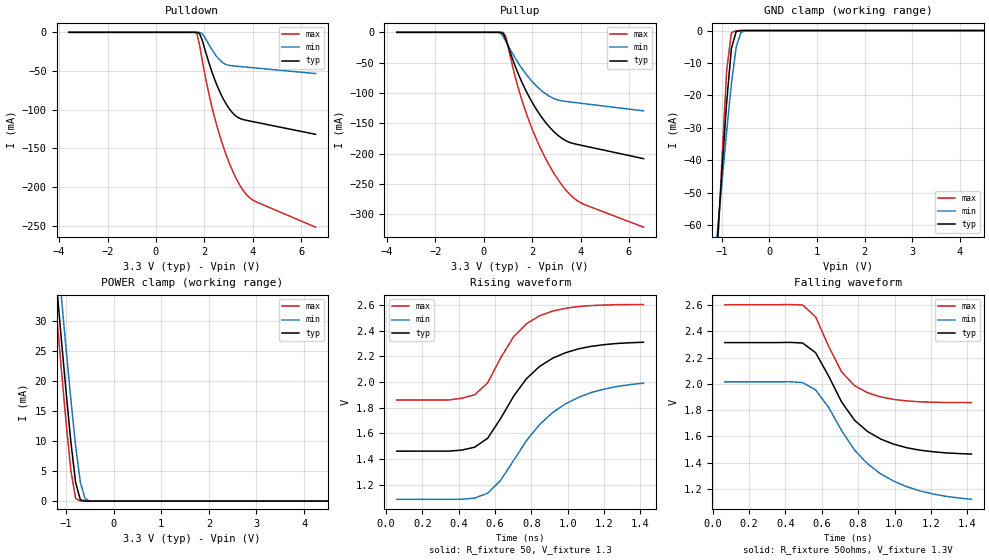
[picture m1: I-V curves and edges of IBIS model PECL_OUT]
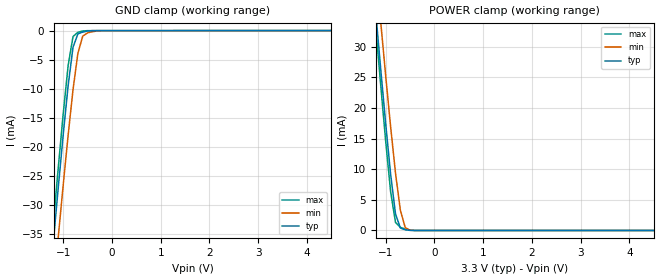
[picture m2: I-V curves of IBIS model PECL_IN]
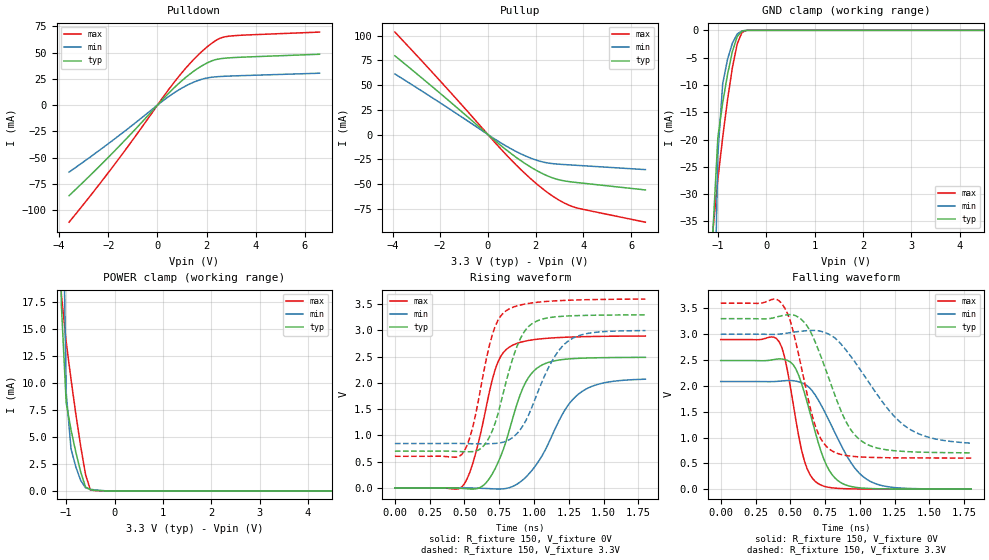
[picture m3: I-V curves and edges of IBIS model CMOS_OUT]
|   This file is an IBIS representation of the   |
|   Texas Instruments   |
|   CDCM1804   |
|   24-pin MLF Package   |
[IBIS Ver]   3.2
[File name]   cdcm1804.ibs
[File Rev]   0.4
[Date]   18th of Feb 2004
[Source]   file originated at Texas Instruments
[Notes]   The following information corresponds to the
|   CDCM1804 i/o buffers and input ESD structures.
|Revision log: 0.1, 06/03/2003 file released by TEXAS INSTRUMENTS.
|   1- initial version
|   0.2, 02/06/2004 file revised for CDCM1804
|   0.3, 02/17/2004 corrected Cin/Cout for PECL outputs,
|   corrected Vinl, Vinh for control input.
|   0.4, 02/18/2004 replaced GND clamp (referenced to VDD) by same
|   plot referenced to GND (0V).
|   Warnings for VT/IV voltage difference relate to truncated
|   VT plots to allow faster simulation frequency if
|   VT time delay is enabled, which is strongly recommended for
|   correct results of the differential PECL buffers. If this is not
|   required, some simulators require to completely disable use of
|   the VT table for better results. If you note problems with
|   differential cross point, it might point to this situation !
[Disclaimer]
(C) Copyright Texas Instruments Incorporated 2004
   All rights reserved
  Texas Instruments Incorporated hereby grants the user of this IBIS
model a non-exclusive, nontransferable license to use this IBIS model
under the following terms.  Before using this IBIS model, the user
should read this license.  If the user does not accept these terms,
the IBIS model should be returned to Texas Instruments within 30 days.
  The user is granted this license only to use the IBIS model and
is not granted rights to sell, load, rent, lease or license the IBIS
model in whole or in part, or in modified form to anyone other than
user.  User may modify the IBIS model to suit its specific applications
but rights to derivative works and such modifications shall belong to
Texas Instruments.
  This IBIS model is provided on an "AS IS" basis and Texas Instruments
makes absolutely no warranty with respect to the information contained
herein.  TEXAS INSTRUMENTS DISCLAIMS AND CUSTOMER WAIVES ALL WARRANTIES,
EXPRESS OR IMPLIED, INCLUDING WARRANTIES OF MERCHANTABILITY OR FITNESS
FOR A PARTICULAR PURPOSE. The entire risk as to quality and performance
is with the Customer. ACCORDINGLY, IN NO EVENT SHALL THE COMPANY BE LIABLE
FOR ANY DAMAGES, WHETHER IN CONTRACT OR TORT,INCLUDING ANY LOST PROFITS
OR OTHER INCIDENTAL, CONSEQUENTIAL, EXEMPLARY, OR PUNITIVE DAMAGES ARISING
OUT OF THE USE OR APPLICATION OF THE IBIS model provided in this package.
Further, Texas Instruments reserves the right to discontinue or make changes
without notice to any product herein to improve reliability, function, or
design. Texas Instruments does not convey any license under patent rights
or any other intellectual property rights, including those of third parties.
Contact Texas Instruments at ATTN: HPA Department,
12500 TI blvd, M/S 8730, Dallas, TX 75243
IBIS Open Forum disclaims all warranties. See DISCLAIM.TXT
in vhdl.org:/pub/IBIS/models for the full disclaimer.
[Copyright]   Copyright 2004, Texas Instruments, All Rights Reserved
[Component]   CDCM1804RTH
[Manufacturer]  Texas Instruments Incorporated
[Package]
|   TYP   MIN   MAX
R_pkg   0.260   0.150   0.310
L_pkg   1.150nH   0.220nH   1.370nH
C_pkg   0.041pF   0.027pF   0.047pF
[Pin]   signal_name   model_name   R_Pin   L_Pin   C_Pin
1   EN   CTRL_IN   0.167ohms   0.683nH   0.028pF
2   VDD   POWER   0.130ohms   0.600nH   0.080pF
3   IN   PECL_IN   0.285ohms   1.249nH   0.044pF
4   INB   PECL_IN   0.270ohms   1.176nH   0.041pF
5   VDD   POWER   0.130ohms   0.600nH   0.080pF
6   VBB   POWER   0.279ohms   1.221nH   0.044pF
7   VSS   GND   0.050ohms   0.220nH   0.240pF
8   VDD   POWER   0.130ohms   0.600nH   0.080pF
9   Y2   PECL_OUT   0.285ohms   1.250nH   0.044pF
10   Y2B   PECL_OUT   0.270ohms   1.177nH   0.041pF
11   VDD   POWER   0.130ohms   0.600nH   0.080pF
12   Y3   CMOS_OUT   0.302ohms   1.331nH   0.045pF
13   VDD   POWER   0.130ohms   0.600nH   0.080pF
14   VDD   POWER   0.130ohms   0.600nH   0.080pF
15   Y1   PECL_OUT   0.270ohms   1.176nH   0.041pF
16   Y1B   PECL_OUT   0.268ohms   1.166nH   0.041pF
17   VDD   POWER   0.130ohms   0.600nH   0.080pF
18   S0   CTRL_IN   0.302ohms   1.331nH   0.045pF
19   S1   CTRL_IN   0.302ohms   1.331nH   0.045pF
20   VDD   POWER   0.130ohms   0.600nH   0.080pF
21   Y0   PECL_OUT   0.270ohms   1.177nH   0.041pF
22   Y0B   PECL_OUT   0.157ohms   0.641nH   0.027pF
23   VDD   POWER   0.130ohms   0.600nH   0.080pF
24   S2   CTRL_IN   0.167ohms   0.683nH   0.028pF
[Diff_Pin]  inv_pin  vdiff   tdelay_typ  tdelay_min  tdelay_max
3   4   0.5V   0ns   0n   0ns   | IN / INB
9   10   0V   0ns   0ns   0ns   | Y2 / Y2B
15   16   0V   0ns   0ns   0ns   | Y1 / Y1B
21   22   0V   0ns   0ns   0ns   | Y0 / Y0B
| Models and submodels in the file (4): PECL_OUT (3-state_ECL), PECL_IN (Input), CMOS_OUT (Output), CTRL_IN (Input)
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|   Differential Output Driver MODEL
[Model]   PECL_OUT
Model_type   3-state_ECL
| Signals   Y0, Y0B, Y1, Y1B, Y2, Y2B,
Vmeas = 1.89V   |Vref for timing measurments
Cref = 0pF   |c_load for timing spec
Rref = 50   |R_load for timing spec
Vref = 1.3V   |Timing spec test load voltage
| variable   typ   min   max
C_comp   0.76pF   NA   NA
[Temperature Range]   27   125   -20
[Voltage range]   3.3V   3.0V   3.6V
[Pulldown reference]   3.3V   3.0V   3.6V
[GND Clamp reference]   0V   0V   0V
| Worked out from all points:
|   GND clamp passes 1 mA (typ) near -0.71 V on its own axis
|   POWER clamp passes 1 mA (typ) near -0.73 V on its own axis
|   rising waveform, R_fixture 50, V_fixture 1.3: 20-80 % time 275ps typ, 321ps min, 209ps max; typ from 1.46 V to 2.31 V
|   falling waveform, R_fixture 50ohms, V_fixture 1.3V: 20-80 % time 251ps typ, 314ps min, 183ps max; typ from 2.31 V to 1.47 V
[Pullup]
|   27C:3.3V:nominal   125C:3.0V:weak   -20C:3.6V:strong
|  Voltage   I(typ)   I(min)   I(max)
-3.6V     437pA      8.06nA     324.7pA
500mV     -84.04nA   -11.65uA   -371.3pA
700mV     -101.2uA   -1.872mA   -2.864uA
800mV     -2.246mA   -7.123mA   -226.3uA
900mV     -11.06mA   -14.21mA   -6.425mA
1.4V      -66.31mA   -49.24mA   -88.69mA
1.9V      -108.6mA   -76.68mA   -149.5mA
2.5V      -146mA     -99.87mA   -204.2mA
3.2V      -174.2mA   -112.9mA   -250.6mA
3.6V      -182.4mA   -115.1mA   -269.2mA
4V        -186.2mA   -117mA     -281.2mA
6.6V      -208.5mA   -129.6mA   -321.5mA
[Pulldown]
|   27C:3.3V:nominal   125C:3.0V:weak   -20C:3.6V:strong
|   Voltage   I(typ)   I(min)   I(max)
-3.6V     280.9pA    304.5pA    264.7pA
1.6V      -1.679uA   -521.3nA   -43.83uA
1.7V      -58.05uA   -8.476uA   -2.396mA
1.8V      -1.47mA    -132uA     -16mA
1.9V      -8.843mA   -1.407mA   -33.6mA
2.2V      -40.32mA   -16.53mA   -81.03mA
2.5V      -66.73mA   -30.89mA   -118.8mA
3V        -97.48mA   -42.66mA   -166.6mA
3.5V      -111.8mA   -44.34mA   -199.5mA
3.8V      -114.3mA   -45.21mA   -211.9mA
4.1V      -116.2mA   -46.08mA   -218.7mA
6.6V      -132mA     -53.32mA   -252.1mA
[GND Clamp]
|   27C:3.3V:nominal   125C:3.0V:weak   -20C:3.6V:strong
|   Voltage   I(typ)   I(min)   I(max)
-3.6V     -846.1mA   -726mA     -1.01A
-1.1V     -65.74mA   -63.12mA   -70.56mA
-1V       -43.58mA   -46.98mA   -40.08mA
-900mV    -22.15mA   -31.16mA   -12.38mA
-800mV    -5.529mA   -16.41mA   -692.9uA
-700mV    -333.5uA   -5.056mA   -8.688uA
-600mV    -9.161uA   -575uA     -94.39nA
-500mV    -237.2nA   -35.55uA   -1.21nA
6.6V      452.4pA    471.7pA    424.6pA
[POWER Clamp]
|   27C:3.3V:nominal   125C:3.0V:weak   -20C:3.6V:strong
|  Voltage   I(typ)   I(min)   I(max)
-3.6V     263.5mA    264.3mA    263.5mA
-1.3V     45.57mA    52.26mA    40.83mA
-1.2V     36.3mA     43.2mA     31.38mA
-1.1V     27.17mA    34.25mA    22.11mA
-1V       18.31mA    25.49mA    13.19mA
-900mV    9.992mA    17.07mA    5.178mA
-800mV    3.144mA    9.308mA    454.2uA
-700mV    228.8uA    3.147mA    5.697uA
-600mV    6.116uA    387.4uA    58.55nA
-500mV    150.9nA    23.42uA    752.7pA
6.6V      0A         0A         0A
[ramp]
| variable   typ   min   max
dV/dt_r   0.5117/2.7842E-10   0.5571/3.3895E-10   0.4456/2.0819E-10
dV/dt_f   0.5117/2.5529E-10   0.5571/3.4568E-10   0.4456/1.8152E-10
[Rising Waveform]
R_fixture = 50
V_fixture =  1.3
V_fixture_min = 1.0
V_fixture_max = 1.6  | Plot was truncated to
|   allow shorter simulation periodes.
|   27C:3.3V:nominal   125C:3.0V:weak  -20C:3.6V:strong
|   Time   V(typ)   V(min)   V(max)
59.71ps   1.462V     1.087V     1.86V
416.9ps   1.47V      1.087V     1.873V
488.3ps   1.492V     1.096V     1.901V
559.7ps   1.562V     1.134V     1.993V
631.1ps   1.716V     1.234V     2.188V
702.6ps   1.89V      1.39V      2.353V
845.4ps   2.121V     1.669V     2.515V
916.9ps   2.185V     1.762V     2.552V
1.06ns    2.258V     1.881V     2.588V
1.417ns   2.31V      1.991V     2.603V
[Falling Waveform]
R_fixture = 50ohms
V_fixture =  1.3V
V_fixture_min = 1.0V
V_fixture_max = 1.6V   |  Plot was truncated to
|   allow shorter simulation periodes.
|   27C:3.3V:nominal   125C:3.0V:weak -20C:3.6V:strong
|   Time   V(typ)   V(min)   V(max)
65.71ps   2.314V     2.015V     2.602V
494.3ps   2.311V     2.01V      2.6V
565.7ps   2.238V     1.955V     2.51V
637.1ps   2.061V     1.822V     2.287V
708.6ps   1.863V     1.645V     2.092V
780ps     1.723V     1.496V     1.987V
922.9ps   1.581V     1.316V     1.901V
1.066ns   1.514V     1.218V     1.87V
1.209ns   1.484V     1.163V     1.86V
1.423ns   1.466V     1.121V     1.858V
|   Differential Input Receiver Model
[Model]   PECL_IN
Model_type   Input
Polarity   Non-Inverting
Enable   Active-High
Vinl = 1.6575V   | PECL levels refer to VDD. 3.3-(1.81+1.475)/2
Vinh = 2.2775V   |   3.3-(1.165+.088)/2
|   typ   min   max
C_comp   0.76pF   NA   NA
[Temperature range]   27   125   -20
[Voltage range]   3.3   3.0   3.6
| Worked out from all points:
|   GND clamp passes 1 mA (typ) near -0.72 V on its own axis
|   POWER clamp passes 1 mA (typ) near -0.73 V on its own axis
| Notes: (1) Vtable = Vcc - Voutput
|   (2) Pullup data includes the effects of the clamping circuitry
[POWER Clamp]
|   27C:3.3V:nominal   125C:3.0V:weak   -20C:3.6V:strong
|  Voltage   I(typ)   I(min)   I(max)
-3.6V     265.8mA    263.4mA    273.1mA
-1.2V     35.02mA    42.56mA    32.64mA
-1.1V     26mA       33.7mA     23.35mA
-1V       17.28mA    25.09mA    14.39mA
-900mV    9.15mA     16.88mA    6.291mA
-800mV    2.691mA    9.338mA    1.306mA
-700mV    397uA      3.282mA    517.8uA
-600mV    106.3uA    454.8uA    227uA
-500mV    15.87uA    36.77uA    48.73uA
6.6V      0A         0A         0A
[GND Clamp]
|   27C:3.3V:nominal   125C:3.0V:weak   -20C:3.6V:strong
|  Voltage   I(typ)   I(min)   I(max)
-3.6V     -268.1mA   -268.4mA   -271.2mA
-1.3V     -45.38mA   -53.26mA   -42.38mA
-1.2V     -35.99mA   -44.19mA   -32.76mA
-1.1V     -26.76mA   -35.23mA   -23.31mA
-1V       -17.81mA   -26.44mA   -14.21mA
-900mV    -9.461mA   -17.98mA   -5.998mA
-800mV    -2.874mA   -10.17mA   -1.017mA
-700mV    -575.1uA   -3.894mA   -292.2uA
-600mV    -252.8uA   -947.5uA   -69.37uA
-500mV    -74.55uA   -385.7uA   -9.282uA
-300mV    -10.26uA   -59.25uA   -7.753uA
6.6V      0A         0A         0A
|   Device Control Output Driver Model
[Model]   CMOS_OUT
Model_type   Output
Polarity   Non-Inverting
Enable   Active-High
Vmeas = 1.65V   |Vref for timing measurements.
Cref = 10pF   |load capacitance for timing spec.
Rref = 500ohms   |1kohm to VCC and 1kohm to GND
Vref = 1.65V   |Timing specification test load voltage; VDD/2
|   typ   min   max
C_comp   1.66pF   NA   NA
[Temperature range]   27   125   -20
[Voltage range]   3.3   3.0   3.6
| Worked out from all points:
|   slope of the pulldown table from 0 to 0.495 V, typ, clamps not added: 40.4 ohm
|   slope of the pullup table from 0 to 0.495 V, typ, clamps not added: 48.6 ohm
|   GND clamp passes 1 mA (typ) near -0.59 V on its own axis
|   POWER clamp passes 1 mA (typ) near -0.65 V on its own axis
|   rising waveform, R_fixture 150, V_fixture 0V: 20-80 % time 192ps typ, 261ps min, 157ps max; typ from 0 V to 2.49 V
|   falling waveform, R_fixture 150, V_fixture 0V: 20-80 % time 167ps typ, 248ps min, 120ps max; typ from 2.49 V to 0.001 V
|   rising waveform, R_fixture 150, V_fixture 3.3V: 20-80 % time 172ps typ, 225ps min, 147ps max; typ from 0.7 V to 3.3 V
|   falling waveform, R_fixture 150, V_fixture 3.3V: 20-80 % time 229ps typ, 351ps min, 157ps max; typ from 3.3 V to 0.704 V
| Notes: (1) Vtable = Vcc - Voutput
|   (2) Pullup data includes the effects of the ESD
|   clamping circuitry
[Pullup]
|   27C:3.3V:nominal   125C:3.0V:weak   -20C:3.6V:strong
|  Voltage   I(typ)   I(min)   I(max)
-3.9V     79.71mA    61.34mA    103.7mA
-1.9V     39.63mA    30.49mA    51.55mA
700mV     -14.19mA   -10.72mA   -18.72mA
1.6V      -30mA      -21.94mA   -40.46mA
2.4V      -40.8mA    -28.27mA   -56.87mA
3V        -45.91mA   -30.04mA   -66.66mA
3.6V      -48.23mA   -30.97mA   -73.35mA
6.6V      -56.06mA   -35.49mA   -88.71mA
[Pulldown]
|   27C:3.3V:nominal   125C:3.0V:weak   -20C:3.6V:strong
|  Voltage   I(typ)   I(min)   I(max)
-3.6V     -86.29mA   -63.84mA   -111.6mA
-2.6V     -63.76mA   -47.12mA   -82.44mA
-1.6V     -40.17mA   -29.64mA   -51.94mA
600mV     14.7mA     10.45mA    19.3mA
1.1V      25.38mA    17.61mA    33.76mA
1.5V      32.68mA    22.09mA    44.06mA
1.9V      38.63mA    25.23mA    53.01mA
2.2V      42.01mA    26.51mA    58.68mA
2.6V      44.31mA    27.3mA     64.14mA
3V        45.14mA    27.73mA    65.87mA
6.6V      48.44mA    30.38mA    69.56mA
[POWER Clamp]
|   27C:3.3V:nominal   125C:3.0V:weak   -20C:3.6V:strong
|  Voltage   I(typ)   I(min)   I(max)
-3.6V     2.308A     2.348A     2.281A
-1.2V     62.21mA    98.1mA     42.9mA
-1.1V     17.3mA     37.08mA    18.26mA
-1V       8.183mA    9.115mA    13.83mA
-900mV    5.658mA    3.897mA    10.35mA
-800mV    3.584mA    2.214mA    7.114mA
-700mV    1.765mA    978.5uA    4.14mA
-600mV    361.7uA    284.9uA    1.527mA
-500mV    114.8uA    158.5uA    94.85uA
-100mV    453.5nA    349.1nA    590.4nA
6.6V      0A         0A         0A
[GND Clamp]
|   27C:3.3V:nominal   125C:3.0V:weak   -20C:3.6V:strong
|  Voltage   I(typ)   I(min)   I(max)
-3.6V     -2.33A     -2.386A    -2.287A
-1.1V     -36.44mA   -65.47mA   -36.48mA
-1V       -19.61mA   -22.75mA   -27.28mA
-900mV    -13.24mA   -9.774mA   -19.6mA
-800mV    -8.089mA   -5.308mA   -12.71mA
-700mV    -3.896mA   -2.367mA   -6.854mA
-600mV    -1.142mA   -668.3uA   -2.488mA
-500mV    -135.2uA   -94.57uA   -356.8uA
-400mV    0A         0A         0A
6.6V      0A         0A         0A
[ramp]
| variable   typ   min   max
| ramp with load to GND
dV/dt_r   1.4917/1.9461E-10   1.2421/2.6550E-10   1.7357/1.5704E-10
| ramp with load to VDD
dV/dt_f   1.5578/2.2888E-10   1.2654/3.5131E-10   1.7979/1.5736E-10
[Rising Waveform]
R_fixture = 150
V_fixture = 0V
|   27C:3.3V:nominal   125C:3.0V:weak  -20C:3.6V:strong
|   Time   V(typ)   V(min)   V(max)
0s        1.549nV    10.29nV    1.008nV
500ps     -12.68mV   1.285mV    80.41mV
580ps     -19.64mV   -3.794mV   654.6mV
680ps     181.8mV    -14.07mV   1.839V
740ps     476.1mV    -21.35mV   2.396V
840ps     1.265V     20.96mV    2.71V
940ps     2.014V     202.9mV    2.797V
1.06ns    2.344V     623.2mV    2.842V
1.34ns    2.47V      1.828V     2.879V
1.8ns     2.486V     2.07V      2.893V
[Falling Waveform]
R_fixture = 150
V_fixture = 0V
|   27C:3.3V:nominal   125C:3.0V:weak  -20C:3.6V:strong
|   Time   V(typ)   V(min)   V(max)
0s        2.49V      2.084V     2.896V
420ps     2.521V     2.09V      2.852V
460ps     2.511V     2.1V       2.546V
520ps     2.412V     2.1V       1.667V
600ps     1.879V     2.037V     559.7mV
700ps     909.2mV    1.732V     108.4mV
820ps     219.1mV    1.097V     20.98mV
940ps     50.26mV    497.5mV    6.743mV
1.06ns    15.02mV    173.4mV    3.081mV
1.8ns     931.8uV    2.188mV    761.4uV
[Rising Waveform]
R_fixture = 150
V_fixture =  3.3V
V_fixture_min = 3.0
V_fixture_max = 3.6
|   27C:3.3V:nominal   125C:3.0V:weak  -20C:3.6V:strong
|   Time   V(typ)   V(min)   V(max)
0s        699.6mV    845.5mV    602.4mV
480ps     691.6mV    845.6mV    634.8mV
560ps     691.4mV    841.1mV    1.163V
660ps     879.2mV    841.2mV    2.492V
720ps     1.231V     847mV      3.072V
800ps     2.029V     890.4mV    3.375V
960ps     3.071V     1.384V     3.513V
1.12ns    3.247V     2.373V     3.557V
1.24ns    3.274V     2.786V     3.573V
1.8ns     3.296V     2.996V     3.596V
[Falling Waveform]
R_fixture = 150
V_fixture =  3.3V
V_fixture_min = 3.0
V_fixture_max = 3.6
|   27C:3.3V:nominal   125C:3.0V:weak  -20C:3.6V:strong
|   Time   V(typ)   V(min)   V(max)
0s        3.3V       3V         3.6V
440ps     3.358V     3.006V     3.588V
500ps     3.38V      3.03V      3.257V
620ps     3.163V     3.068V     1.849V
700ps     2.708V     3.066V     1.083V
800ps     1.972V     2.965V     740.9mV
920ps     1.213V     2.624V     644.7mV
1.06ns    857.5mV    2.085V     617.5mV
1.36ns    724.9mV    1.159V     605.5mV
1.8ns     703.7mV    890.9mV    603.4mV
